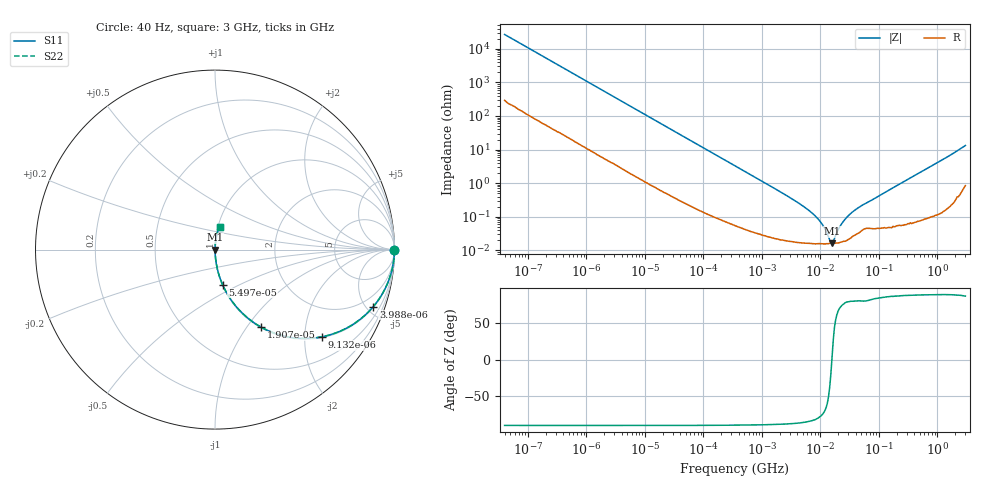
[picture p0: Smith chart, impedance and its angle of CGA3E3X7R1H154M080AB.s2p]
! S-parameter Generated by TDK Corporation
! Copyright(C) 2015 TDK Corporation.
! All Rights Reserved.
! TDK P/N: CGA3E3X7R1H154M080AB (Multilayer Ceramic Chip Capacitors)
! Property: C=150nF
! Size(LxWxT): 1.6x0.8x0.8mm, 0.063x0.031x0.031inches
! Model Type: s2p (Touchstone File Format Version 1.0)
! Frequency: DC=Yes Start=0.00004MHz Stop=3000MHz 396points Log-sweep
! Note: This model was converted from impedance.
! Model Generated on Jun. 23, 2015
! Hash(MD5):
! Port Assignments:
!  1 ---| |--- 2
! Applicable Conditions:
!  Temperature = 25 degC
!  DC Bias Voltage = 0 V
!  Small Signal Operation
! Terms and conditions regarding TDK Simulation Models
! (1)This simulation model is being provided solely for informational purposes. Please refer to the specifications of the products in terms of detailed characteristics of such products.
! (2)In no event shall TDK Corporation of any of its subsidiaries be liable for any loss or damage arising, directly or indirectly,
!  From any information contained in this simulation model, including, but not limited to loss or damages arising from any inaccuracies, omissions or errors in connection with such information.
! (3)Any and all copyrights on this simulation model are owned by TDK Corporation.
!  Duplication or redistribution of this simulation model without prior written permission from TDK Corporation is prohibited.
! (4)This simulation model is subject to any modification or change without any prior notice.
! (5)Neither TDK Corporation nor any of its subsidiaries shall make any warranty, express or implied,
!  Including but not limited to the correctness, implied warranties of merchantability and fitness for a particular purpose with respect to this simulation models.
! (6)The use of this simulation model shall be deemed to have consented to the terms and conditions hereof.
# MHz S MA R 50
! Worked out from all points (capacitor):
!   395 points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, 40 Hz to 3 GHz, reference 50 ohm
!   read as one part in series: C = 148 nF near 41.88 Hz
!   lowest |Z| = 16.4 mohm at 15.8 MHz (marker M1)
!   series resonance near 15.67 MHz, so ESL is about 700 pH
!   S11 on the Smith chart (normalised r, x): 40 Hz: open; 3.988 kHz: 1.05, -5.53; 9.132 kHz: 1.02, -2.43; 19.07 kHz: 1.01, -1.17; 54.97 kHz: 1.00, -0.41; 3 GHz: 1.02, +0.26
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4e-05  1 -0.2  0.003737 89.2  0.003737 89.2  1 -0.2
0.000834128  0.9964 -4.4  0.07605 85.1  0.07605 85.1  0.9964 -4.4
0.001909884  0.9836 -9.8  0.171 79.6  0.171 79.6  0.9836 -9.8
0.003988472  0.9375 -19.8  0.3389 69.6  0.3389 69.6  0.9375 -19.8
0.009132315  0.7683 -39.2  0.6326 50.2  0.6326 50.2  0.7683 -39.2
0.01739424  0.5366 -57.0  0.8385 32.4  0.8385 32.4  0.5366 -57.0
0.0190713  0.5022 -59.3  0.8597 30.1  0.8597 30.1  0.5022 -59.3
0.03164043  0.332 -70.0  0.9398 19.4  0.9398 19.4  0.332 -70.0
0.05496573  0.1998 -77.8  0.9776 11.5  0.9776 11.5  0.1998 -77.8
0.3464102  0.03293 -87.2  0.9989 1.9  0.9989 1.9  0.03293 -87.2
2.748062  0.004111 -87.1  0.9998 0.2  0.9998 0.2  0.004111 -87.1
7.22376  0.001284 -82.8  0.9998 0.1  0.9998 0.1  0.001284 -82.8
10.93076  0.0005691 -73.9  0.9998 0.0  0.9998 0.0  0.0005691 -73.9
12.54911  0.0003704 -64.6  0.9998 0.0  0.9998 0.0  0.0003704 -64.6
15.08561  0.000173 -19.1  0.9998 0.0  0.9998 0.0  0.000173 -19.1
15.79611  0.0001638 4.2  0.9998 -0.0  0.9998 -0.0  0.0001638 4.2
21.8003  0.0005371 71.1  0.9998 -0.0  0.9998 -0.0  0.0005371 71.1
31.50375  0.001171 79.0  0.9998 -0.1  0.9998 -0.1  0.001171 79.0
52.26661  0.002232 79.5  0.9996 -0.1  0.9996 -0.1  0.002232 79.5
150.6385  0.006348 85.3  0.9995 -0.4  0.9995 -0.4  0.006348 85.3
1040.901  0.04266 86.0  0.9979 -2.4  0.9979 -2.4  0.04266 86.0
3000  0.1305 78.9  0.9832 -7.5  0.9832 -7.5  0.1305 78.9
